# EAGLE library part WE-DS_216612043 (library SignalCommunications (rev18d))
WE-DS D-SUB-Filter Connectors Bent 90° Characteristics Standard type filtered with 1000 pF High attenuation of more than 40 dB @ 180 MHz Choice of earthing metal sheet or high speed earthing clip Rated voltage: 100 VDC Rated current @ 20 ºC: 5 A Withstand voltage: 250 VRMS Insulation resistance: min. 1000 MΩ Operating temperature: –55 ºC to +125 ºC Applications Filtering of interfaces External connection to -printer -sensor -display Details see: http://katalog.we-online.de/en/pbs/Filter_abgewinkelt Created on 2015-05-04 2015 (C) Wurth Elektronik
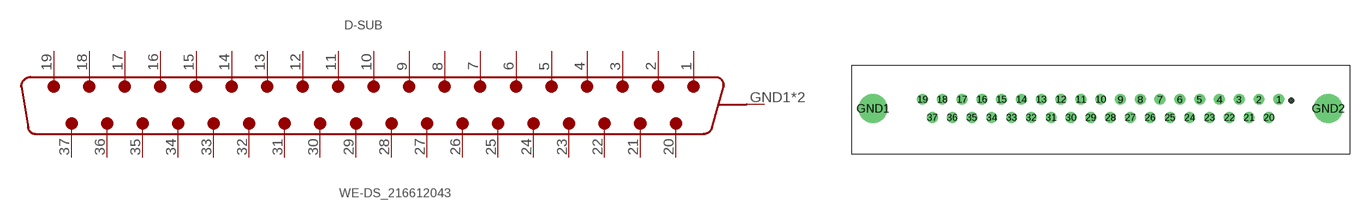
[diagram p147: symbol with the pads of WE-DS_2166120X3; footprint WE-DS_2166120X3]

Designator prefix D-SUB

## WE-DS_216612043 (WE-NUMBER: 216612043/37pins_female)  [WE-DS_2166120X3]
1  19  pas
2  18  pas
3  17  pas
4  16  pas
5  15  pas
6  14  pas
7  13  pas
8  12  pas
9  11  pas
10  10  pas
11  9  pas
12  8  pas
13  7  pas
14  6  pas
15  5  pas
16  4  pas
17  3  pas
18  2  pas
19  1  pas
20  37  pas
21  36  pas
22  35  pas
23  34  pas
24  33  pas
25  32  pas
26  31  pas
27  30  pas
28  29  pas
29  28  pas
30  27  pas
31  26  pas
32  25  pas
33  24  pas
34  23  pas
35  22  pas
36  21  pas
37  20  pas
GND1  GND  pwr
GND2  GND  pwr

## Footprint WE-DS_2166120X3 (pad centres in mm)
drill 1: 1 24.84,1.27; 2 22.1,1.27; 3 19.33,1.27; 4 16.56,1.27; 5 13.82,1.27; 6 11.05,1.27; 7 8.28,1.27; 8 5.54,1.27; 9 2.77,1.27; 10 0,1.27; 11 -2.77,1.27; 12 -5.54,1.27; 13 -8.28,1.27; 14 -11.05,1.27; 15 -13.82,1.27; 16 -16.56,1.27; 17 -19.33,1.27; 18 -22.1,1.27; 19 -24.84,1.27; 20 23.47,-1.27; 21 20.7,-1.27; 22 17.96,-1.27; 23 15.19,-1.27; 24 12.42,-1.27; 25 9.68,-1.27; 26 6.91,-1.27; 27 4.14,-1.27; 28 1.38,-1.27; 29 -1.38,-1.27; 30 -4.14,-1.27; 31 -6.91,-1.27; 32 -9.68,-1.27; 33 -12.42,-1.27; 34 -15.19,-1.27; 35 -17.96,-1.27; 36 -20.7,-1.27; 37 -23.47,-1.27
drill 3: GND1 -31.75,0; GND2 31.75,0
